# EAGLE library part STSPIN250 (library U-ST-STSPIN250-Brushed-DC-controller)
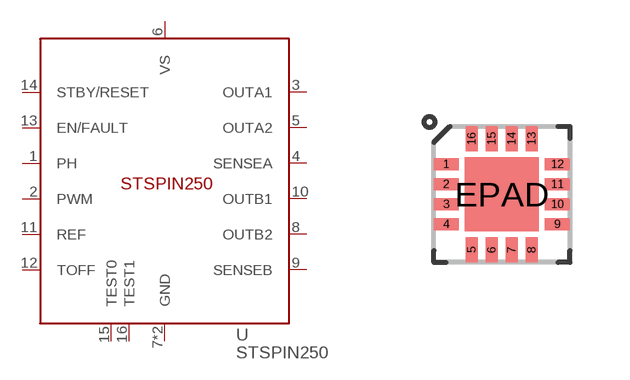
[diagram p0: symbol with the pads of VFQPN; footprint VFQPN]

Designator prefix U

## STSPIN250  [VFQPN]
1  PH  in
2  PWM  in
3  OUTA1  out
4  SENSEA  out
5  OUTA2  out
6  VS  pwr
7  GND  pwr
8  OUTB2  out
9  SENSEB  out
10  OUTB1  out
11  REF  pas
12  TOFF  pas
13  EN/FAULT
14  STBY/RESET
15  TEST0
16  TEST1
EPAD  GND  pwr

## Footprint VFQPN (pad centres in mm)
smd 0.63 x 0.3: 1 -1.39,0.75; 2 -1.39,0.25; 3 -1.39,-0.25; 4 -1.39,-0.75; 9 1.39,-0.75; 10 1.39,-0.25; 11 1.39,0.25; 12 1.39,0.75
smd 0.3 x 0.63: 5 -0.75,-1.39; 6 -0.25,-1.39; 7 0.25,-1.39; 8 0.75,-1.39; 13 0.75,1.39; 14 0.25,1.39; 15 -0.25,1.39; 16 -0.75,1.39
smd 1.85 x 1.85: EPAD 0,0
